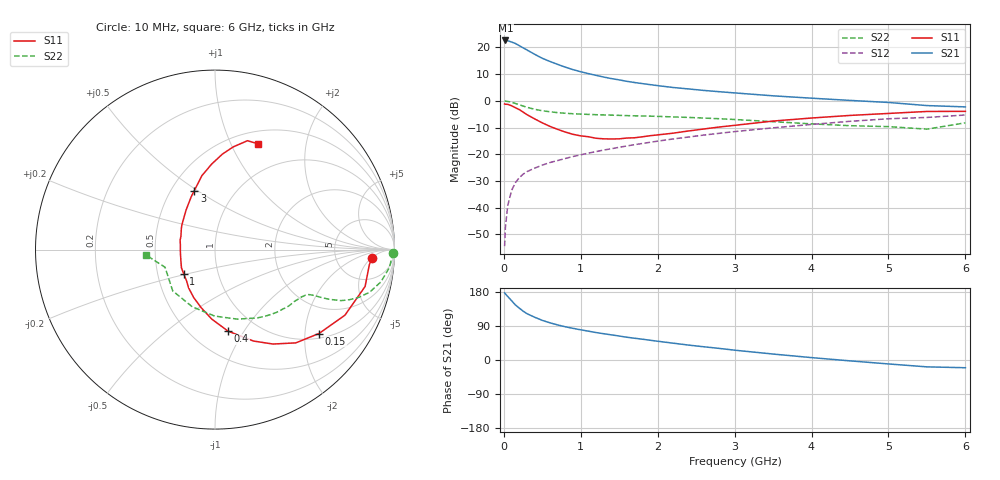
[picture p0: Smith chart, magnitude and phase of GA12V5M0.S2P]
! Infineon Technologies  Discrete & RF Semiconductors
! BF775
! Si NPN RF Bipolar Junction Transistor in SOT23
! VCE = 12 V  IC = 5 mA
! Common Emitter S-Parameters:  May  1996
# GHz  S  MA  R  50
!  f  S11  S21  S12  S22
! GHz  MAG  ANG  MAG  ANG  MAG  ANG  MAG  ANG
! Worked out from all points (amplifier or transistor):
!   36 points, 10 MHz to 6 GHz, reference 50 ohm
!   highest |S21| = 22.6 dB at 20 MHz (marker M1)
!   |S21| within 3 dB of that: start of sweep to 265.3 MHz
!   unconditionally stable (mu >= 1): 870.8 MHz to 2.87 GHz
!   at 250 MHz: K = 0.47, MSG = 23.7 dB, |S12| = -27.5 dB
!   at 1.4 GHz: K = 1.10, MAG = 11.2 dB, |S12| = -17.9 dB
!   at 6 GHz: K = 0.87, MSG = 1.5 dB, |S12| = -5.3 dB
!   S11 on the Smith chart (normalised r, x): 10 MHz: 13, -5; 150 MHz: 1.13, -2.36; 400 MHz: 0.74, -0.85; 1 GHz: 0.68, -0.20; 3 GHz: 0.65, +0.49; 6 GHz: 0.65, +1.28
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0.01  0.8761 -2.9  13.49 177.1  0.0019 83.2  0.9913 -1.0
0.02  0.864 -5.6  13.52 174.5  0.0042 84.3  0.9872 -2.4
0.05  0.8612 -13.8  13.35 167.7  0.0108 81.3  0.9769 -5.9
0.1  0.8109 -26.8  12.65 156.6  0.0209 76.2  0.9417 -11.0
0.15  0.7444 -38.9  11.88 145.3  0.0293 69.9  0.894 -15.4
0.2  0.6876 -49.1  10.81 137.0  0.0363 65.7  0.8457 -18.3
0.25  0.6171 -58.5  9.845 129.1  0.0423 62.7  0.8004 -20.4
0.3  0.5525 -67.2  8.986 122.4  0.0472 61.1  0.7588 -22.0
0.4  0.4601 -80.9  7.456 112.9  0.0549 59.0  0.695 -23.5
0.5  0.3874 -92.7  6.273 104.6  0.0626 58.2  0.6527 -24.2
0.6  0.3322 -103.5  5.463 98.1  0.07 58.0  0.6244 -24.6
0.7  0.2925 -113.9  4.818 92.5  0.0763 58.7  0.6015 -25.0
0.8  0.2602 -124.2  4.273 87.6  0.0834 58.8  0.5858 -25.4
1  0.2208 -141.9  3.507 79.6  0.0976 59.6  0.5649 -26.6
1.1  0.2128 -151.5  3.236 76.1  0.1051 60.0  0.5579 -27.7
1.6  0.2013 164.8  2.321 60.0  0.1431 59.9  0.529 -32.9
2.2  0.2481 134.3  1.78 44.4  0.1934 57.8  0.5003 -41.9
3  0.3479 109.4  1.409 25.9  0.2657 51.9  0.4477 -58.2
3.5  0.4188 100.0  1.242 15.7  0.3124 47.0  0.4072 -72.1
4.5  0.5333 85.6  1.02 -2.3  0.4139 35.7  0.3427 -111.8
5.5  0.6331 73.4  0.816 -18.1  0.4892 20.2  0.2952 -160.5
6  0.6365 67.7  0.771 -20.4  0.5436 15.9  0.3877 -175.8
